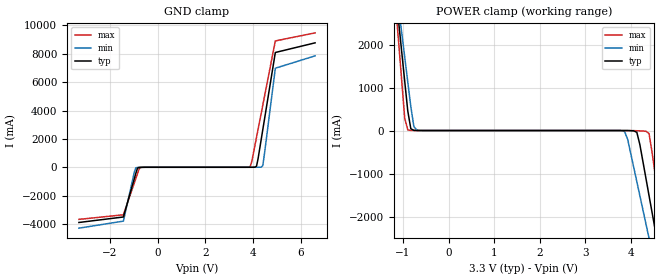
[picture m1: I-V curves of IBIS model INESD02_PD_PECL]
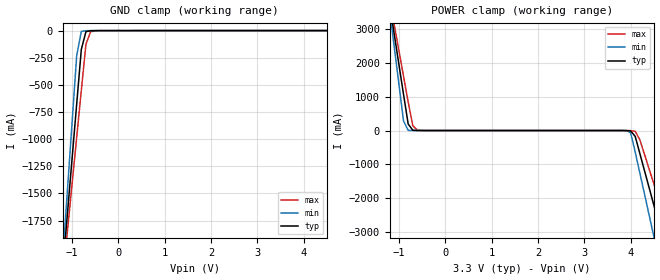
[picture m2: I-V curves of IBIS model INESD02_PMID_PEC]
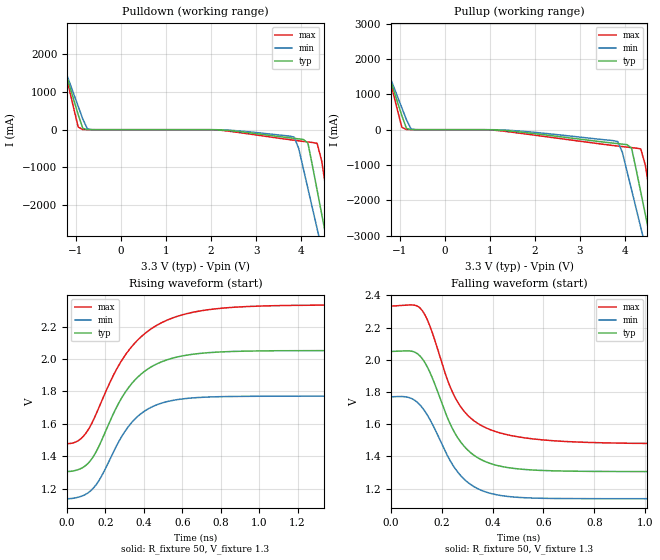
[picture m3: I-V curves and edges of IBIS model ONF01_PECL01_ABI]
|   This file is an IBIS representation of the   |
|   Integrated Devices Technology, Inc.   |
|   ICS873991   |
|   LOW VOLTAGE, LVCMOS/CRYSTAL-TO-LVPECL/ECL CLOCK GENERATOR   |
[IBIS Ver]   4.1
[File name]   873991_3v3.ibs
[File Rev]   1.0
[Date]   24 Dec 2008 | Last modified
[Source]   Originated at Integrated Devices Technology, Inc.
[Disclaimer]
IDT hereby grants the user of this IBIS model a non-exclusive,
nontransferable license to use this IBIS model under the following terms.
Before using this IBIS model, the user should read this license.
If the user does not accept these terms,  the IBIS model should be
returned to IDT within 30 days.
   The user is granted this license only to use the IBIS model and
is not granted rights to sell, load, rent, lease or license the IBIS
model in whole or in part, or in modified form to anyone other than
user. User may modify the IBIS model to suit its specific
applications but rights to derivative works and such modifications
shall belong to IDT.
   This IBIS model is provided on an "AS IS" basis and IDT makes
absolutely no warranty with respect to the information contained
herein. IDT DISCLAIMS AND CUSTOMER WAIVES ALL WARRANTIES, EXPRESS
OR IMPLIED, INCLUDING WARRANTIES OF MERCHANTABILITY OR FITNESS FOR
A PARTICULAR PURPOSE. The entire risk as to quality and performance
is with the Customer. ACCORDINGLY, IN NO EVENT SHALL THE COMPANY BE
LIABLE FOR ANY DAMAGES, WHETHER IN CONTRACT OR TORT,INCLUDING ANY
LOST PROFITS OR OTHER INCIDENTAL, CONSEQUENTIAL, EXEMPLARY, OR
PUNITIVE DAMAGES ARISING OUT OF THE USE OR APPLICATION OF THE IBIS
model provided in this package. Further, IDT reserves the right to
make changes without notice to any product herein to improve
reliability, function, or design. IDT does not convey any license
under patent rights or any other intellectual property rights,
including those of third parties.
   IDT is not obligated to provide maintenance or support
for the licensed IBIS model.
[Copyright]   Copyright 2004 by Integrated Devices Technology, Inc.
[Component]   ICS873991
[Manufacturer] Integrated Devices Technology, Inc.
[Package]
|LQFP 52 Pin
|   typ   min   max
R_pkg   52.85m   52.5m   53.2m
L_pkg   3.26nH   2.86nH   3.66nH
C_pkg   0.487pF   0.443pF   0.53pF
[Pin]   signal_name   model_name   R_pin   L_pin   C_pin
1   VEE   GND   53.20m   3.66n   0.530p
2   MR   INESD02_PD_PECL   53.08m   3.53n   0.523p
3   PLL_EN   INESD02_PD_PECL   52.97m   3.39n   0.516p
4   REF_SEL   INESD02_PD_PECL   52.85m   3.26n   0.509p
5   FSEL_FB2   INESD02_PD_PECL   52.73m   3.13n   0.501p
6   FSEL_FB1   INESD02_PD_PECL   52.62m   2.99n   0.494p
7   FSEL_FB0   INESD02_PD_PECL   52.50m   2.86n   0.487p
8   TEST_CLK   INESD02_PD_PECL   52.62m   2.99n   0.494p
9   PCLK   INESD02_PD_PECL   52.73m   3.13n   0.501p
10   nPCLK   INESD02_PMID_PEC   52.85m   3.26n   0.509p
11   VCC   POWER   52.97m   3.39n   0.516p
12   EXT_FB   INESD02_PD_PECL   53.08m   3.53n   0.523p
13   nEXT_FB   INESD02_PMID_PEC   53.20m   3.66n   0.530p
14   VCCA   POWER   53.20m   3.66n   0.530p
15   nQFB   ONF01_PECL01_ABI   53.08m   3.53n   0.523p
16   QFB   ONF01_PECL01_ABI   52.97m   3.39n   0.516p
17   VCCO   POWER   52.85m   3.26n   0.509p
18   nQD0   ONF01_PECL01_ABI   52.73m   3.13n   0.501p
19   QD0   ONF01_PECL01_ABI   52.62m   2.99n   0.494p
20   nQD1   ONF01_PECL01_ABI   52.50m   2.86n   0.487p
21   QD1   ONF01_PECL01_ABI   52.62m   2.99n   0.494p
22   VCCO   POWER   52.73m   3.13n   0.501p
23   nQC0   ONF01_PECL01_ABI   52.85m   3.26n   0.509p
24   QC0   ONF01_PECL01_ABI   52.97m   3.39n   0.516p
25   nQC1   ONF01_PECL01_ABI   53.08m   3.53n   0.523p
26   QC1   ONF01_PECL01_ABI   53.20m   3.66n   0.530p
27   FSEL3   INESD02_PD_PECL   53.20m   3.66n   0.530p
28   nQC2   ONF01_PECL01_ABI   53.08m   3.53n   0.523p
29   QC2   ONF01_PECL01_ABI   52.97m   3.39n   0.516p
30   VCCO   POWER   52.85m   3.26n   0.509p
31   nQB0   ONF01_PECL01_ABI   52.73m   3.13n   0.501p
32   QB0   ONF01_PECL01_ABI   52.62m   2.99n   0.494p
33   FSEL2   INESD02_PD_PECL   52.50m   2.86n   0.487p
34   nQB1   ONF01_PECL01_ABI   52.62m   2.99n   0.494p
35   QB1   ONF01_PECL01_ABI   52.73m   3.13n   0.501p
36   FSEL1   INESD02_PD_PECL   52.85m   3.26n   0.509p
37   nQB2   ONF01_PECL01_ABI   52.97m   3.39n   0.516p
38   QB2   ONF01_PECL01_ABI   53.08m   3.53n   0.523p
39   FSEL0   INESD02_PD_PECL   53.20m   3.66n   0.530p
40   nQB3   ONF01_PECL01_ABI   53.20m   3.66n   0.530p
41   QB3   ONF01_PECL01_ABI   53.08m   3.53n   0.523p
42   VCCO   POWER   52.97m   3.39n   0.516p
43   nQA0   ONF01_PECL01_ABI   52.85m   3.26n   0.509p
44   QA0   ONF01_PECL01_ABI   52.73m   3.13n   0.501p
45   nQA1   ONF01_PECL01_ABI   52.62m   2.99n   0.494p
46   QA1   ONF01_PECL01_ABI   52.50m   2.86n   0.487p
47   nQA2   ONF01_PECL01_ABI   52.62m   2.99n   0.494p
48   QA2   ONF01_PECL01_ABI   52.73m   3.13n   0.501p
49   nQA3   ONF01_PECL01_ABI   52.85m   3.26n   0.509p
50   QA3   ONF01_PECL01_ABI   52.97m   3.39n   0.516p
51   SYNC_SEL   INESD02_PD_PECL   53.08m   3.53n   0.523p
52   VCO_SEL   INESD02_PD_PECL   53.20m   3.66n   0.530p
[Diff Pin]  inv_pin  vdiff tdelay_typ tdelay_min  tdelay_max
|Output
16   15   NA   0   0   0
19   18   NA   0   0   0
21   20   NA   0   0   0
24   23   NA   0   0   0
26   25   NA   0   0   0
29   28   NA   0   0   0
32   31   NA   0   0   0
35   34   NA   0   0   0
38   37   NA   0   0   0
41   40   NA   0   0   0
44   43   NA   0   0   0
46   45   NA   0   0   0
48   47   NA   0   0   0
50   49   NA   0   0   0
|Input
9   10   0.3   0   0   0
12   13   0.3   0   0   0
| Models and submodels in the file (3): INESD02_PD_PECL (Input), INESD02_PMID_PEC (Input), ONF01_PECL01_ABI (Output_ECL)
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[Model]   INESD02_PD_PECL
Model_type  Input
Polarity   Non-Inverting
Vinl = 0.8V
Vinh = 2.0V
|   typ   min   max
C_comp   2pF   1.5pF   2.5pF
|   typ   min   max
[Voltage range]  3.3V   3.15V   3.45V
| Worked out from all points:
|   GND clamp passes 1 mA (typ) near -0.59 V on its own axis
|   POWER clamp passes 1 mA (typ) near -0.70 V on its own axis
[GND_clamp]
-3.3V     -3.894A    -4.294A    -3.674A
-1.434V   -3.506A    -3.799A    -3.352A
-974.8mV  -794.1mA   -331.5mA   -1.096A
-909.1mV  -407.1mA   -35.25mA   -774.3mA
-777.8mV  -10.55mA   -10.84mA   -133.1mA
-646.5mV  -1.912mA   -4.151mA   -2.665mA
3.884V    141.8uA    72.03uA    57.99mA
3.95V     342.2uA    75.94uA    423.8mA
4.146V    78.32mA    440.9uA    2.118A
4.409V    2.651A     112.4mA    4.38A
4.934V    8.093A     6.984A     8.908A
6.6V      8.773A     7.854A     9.475A
[POWER_clamp]
-3.3V     6.7A       6.327A     7.39A
-1.165V   3.23A      3.44A      2.951A
-1.031V   1.843A     2.286A     1.176A
-963.9mV  1.149A     1.709A     289.6mA
-896.9mV  456.5mA    1.133A     15.4mA
-695.9mV  792.2uA    10.73mA    555.6uA
3.861V    -556.7uA   -26.14mA   -39.45uA
4.129V    -41.85mA   -1.19A     -4.904mA
4.33V     -1.119A    -2.176A    -17.86mA
4.531V    -2.305A    -3.163A    -1.019A
4.732V    -3.492A    -4.151A    -2.536A
6.6V      -5.075A    -5.468A    -4.558A
[Model]   INESD02_PMID_PEC
Model_type   Input
Polarity   Non-Inverting
Vinl = 0.8V
Vinh = 2.0V
|   typ   min   max
C_comp   2pF   1.5pF   2.5pF
|   typ   min   max
[Voltage range]  3.3V   3.15V   3.45V
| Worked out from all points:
|   GND clamp passes 1 mA (typ) near -0.54 V on its own axis
|   POWER clamp passes 1 mA (typ) near -0.60 V on its own axis
[GND_clamp]
|Voltage   I(typ)   I(min)   I(max)
-3.3V     -12.83A    -15.14A    -11.37A
-1.2V     -2.195A    -2.092A    -2.281A
-1.1V     -1.689A    -1.472A    -1.849A
-900mV    -678.6mA   -232.7mA   -984.9mA
-800mV    -174mA     -7.255mA   -553.3mA
-700mV    -9.789mA   -1.13mA    -126.1mA
-600mV    -1.72mA    -254.4uA   -11.17mA
-500mV    -427uA     -99.72uA   -2.216mA
6.6V      76.52uA    70.16uA    79.2uA
[POWER_clamp]
|Voltage   I(typ)   I(min)   I(max)
-3.3V     22.38A     26.45A     19.82A
-1.2V     3.723A     3.545A     3.874A
-1.1V     2.836A     2.457A     3.116A
-900mV    1.063A     281mA      1.601A
-800mV    191.6mA    5.071mA    844mA
-600mV    678.1uA    76.63uA    10.7mA
3.9V      -1.629mA   -3.157mA   -831.1uA
4.1V      -173.9mA   -635.2mA   -23.94mA
4.5V      -2.195A    -3.116A    -1.568A
4.7V      -3.206A    -4.358A    -2.433A
4.9V      -4.218A    -5.6A      -3.298A
6.6V      -12.83A    -16.16A    -10.66A
[Model]   ONF01_PECL01_ABI
Model_type  Output_ECL
Polarity   Non-Inverting
Vmeas = 1.63
Rref = 50
Cref = 0
Vref = 1.3
|Variable  typ   min   max
C_comp   2p   1.5p   2.5p
[Voltage Range]   3.3   3.135   3.465
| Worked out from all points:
|   rising waveform, R_fixture 50, V_fixture 1.3: 20-80 % time 218ps typ, 193ps min, 263ps max; typ from 1.31 V to 2.05 V
|   falling waveform, R_fixture 50, V_fixture 1.3: 20-80 % time 134ps typ, 136ps min, 142ps max; typ from 2.05 V to 1.31 V
| Open source, no load
|  Voltage   I(typ)   I(min)   I(max)
[Pulldown]
-3.3V     9.786A     8.425A     12.06A
-1.667V   3.247A     2.986A     3.704A
-1.463V   2.432A     2.308A     2.661A
-952.6mV  398mA      618.5mA    68.87mA
-850.5mV  36.63mA    281.6mA    4.032mA
3.844V    -229.1mA   -195.7mA   -279.4mA
4.151V    -352.7mA   -1.559A    -324.9mA
4.355V    -1.599A    -2.62A     -360.9mA
4.559V    -2.871A    -3.681A    -1.635A
4.661V    -3.508A    -4.211A    -2.446A
4.763V    -4.144A    -4.742A    -3.257A
6.6V      -15.69A    -14.35A    -17.99A
[Pullup]
-3.3V     9.786A     8.425A     12.06A
-1.565V   2.839A     2.647A     3.182A
-952.6mV  398mA      618.5mA    68.87mA
-850.5mV  36.63mA    281.6mA    4.032mA
-646.4mV  229.3uA    964.8uA    177.5uA
3.844V    -394.4mA   -337mA     -463.1mA
4.151V    -517.8mA   -1.701A    -507.4mA
4.355V    -1.764A    -2.763A    -542.7mA
4.559V    -3.036A    -3.825A    -1.816A
4.661V    -3.672A    -4.355A    -2.626A
4.763V    -4.308A    -4.886A    -3.437A
6.6V      -15.79A    -14.46A    -18.06A
[Ramp]
|   typ   min   max
dV/dt_r   0.596/0.354n   0.506/0.311n   0.684/0.427n
dV/dt_f   0.599/0.219n   0.507/0.219n   0.690/0.252n
R_load =   50.0000
[Rising Waveform]
R_fixture = 50
V_fixture = 1.3   | VCC_typ - 2V
V_fixture_max = 1.465   | VCC_max - 2V
V_fixture_min = 1.135   | VCC_min - 2V
C_fixture = 0.0p
| Time   typ   min   max
0s        1.306V     1.138V     1.478V
67.2ps    1.321V     1.15V      1.503V
126ps     1.379V     1.19V      1.597V
176.4ps   1.489V     1.271V     1.731V
247.8ps   1.679V     1.442V     1.915V
338.1ps   1.85V      1.61V      2.079V
430.5ps   1.946V     1.698V     2.18V
554.4ps   2.007V     1.745V     2.255V
936.6ps   2.049V     1.77V      2.324V
1.999ns   2.052V     1.771V     2.333V
[Falling Waveform]
R_fixture = 50
V_fixture = 1.3   | VCC_typ - 2V
V_fixture_max = 1.465   | VCC_max - 2V
V_fixture_min = 1.135   | VCC_min - 2V
C_fixture = 0.0p
| Time   typ   min   max
0s        2.052V     1.771V     2.334V
73.5ps    2.055V     1.765V     2.34V
119.7ps   2.015V     1.711V     2.314V
151.2ps   1.932V     1.637V     2.221V
224.7ps   1.633V     1.399V     1.868V
268.8ps   1.503V     1.293V     1.723V
336ps     1.398V     1.205V     1.611V
434.7ps   1.338V     1.157V     1.544V
806.4ps   1.307V     1.138V     1.486V
1.999ns   1.306V     1.138V     1.478V
